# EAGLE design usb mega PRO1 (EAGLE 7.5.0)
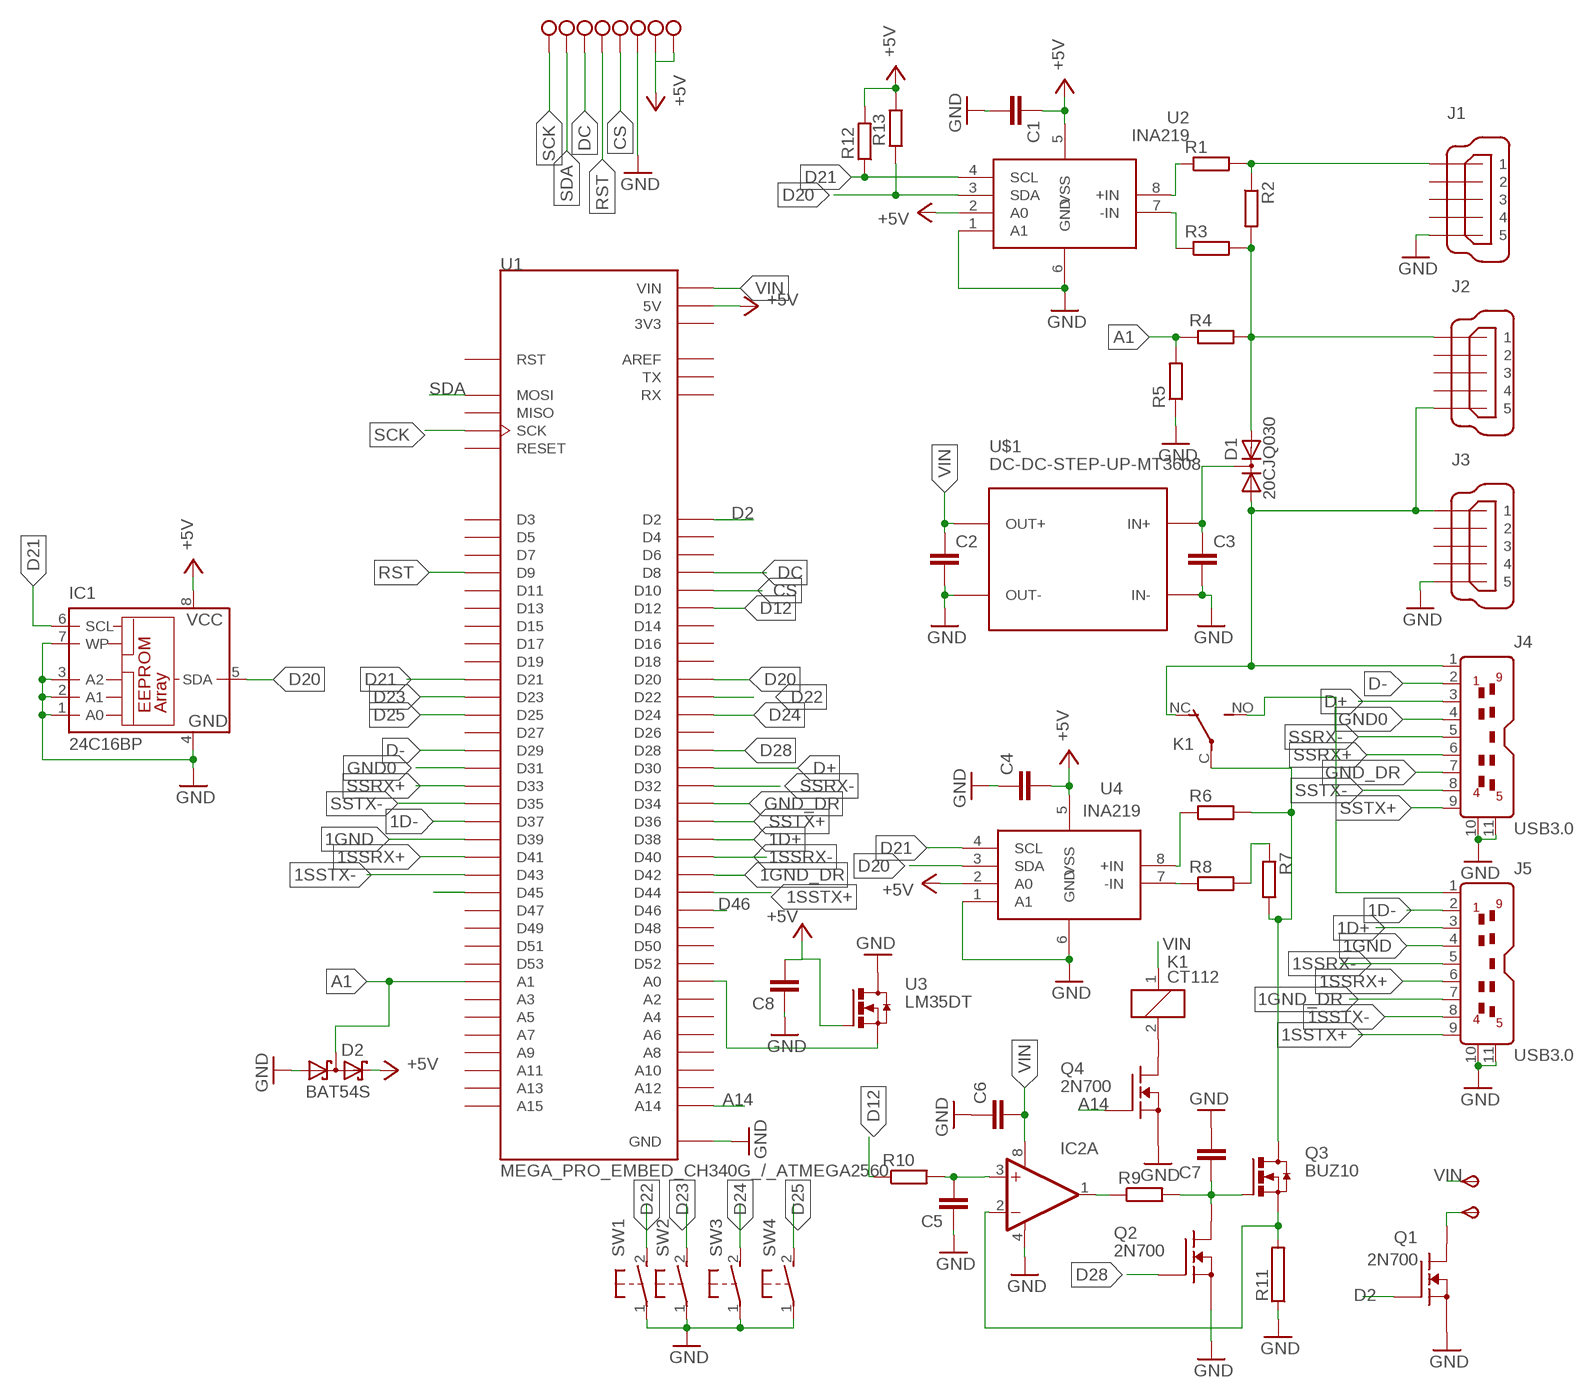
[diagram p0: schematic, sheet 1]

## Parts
C1  C-EUC0805  [C0805]
C2  C-EUC1206  [C1206]
C3  C-EUC1206  [C1206]
C4  C-EUC0805  [C0805]
C5  C-EUC0805  [C0805]
C6  C-EUC0805  [C0805]
C7  C-EUC0805  [C0805]
C8  C-EUC1206  [C1206]
D1  20CJQ030  [SOT223]
D2  BAT54S  [SOT23]
IC1  24C16BP  [DIL8]
IC2  OPA2658U  [SO08]
J1  MINI-USB_SHIELD5P2-32005-601  [32005-601]
J2  MINI-USB_SHIELD5P2-32005-601  [32005-601]
J3  MINI-USB_SHIELD5P2-32005-601  [32005-601]
J4  USB3.0  [USB3.0]
J5  USB3.0  [USB3.0]
K1  CT112  [CT-SLIM]
Q1  2N700  BSS138  [SOT23]
Q2  2N700  BSS138  [SOT23]
Q3  BUZ10  [TO220MIRROR]
Q4  2N700  BSS138  [SOT23]
R1  R-EU_R0805  [R0805]
R2  R-EU_R2010  [R2010]
R3  R-EU_R0805  [R0805]
R4  R-EU_R0805  [R0805]
R5  R-EU_R0805  [R0805]
R6  R-EU_R0805  [R0805]
R7  R-EU_R2010  [R2010]
R8  R-EU_R0805  [R0805]
R9  R-EU_R0805  [R0805]
R10  R-EU_R0805  [R0805]
R11  RAC01  [AC01]
R12  R-EU_R0805  [R0805]
R13  R-EU_R0805  [R0805]
SCK  TP2P2-38-17  [P2-38-17]
SCK1  TP2P2-38-17  [P2-38-17]
SCK2  TP2P2-38-17  [P2-38-17]
SCK3  TP2P2-38-17  [P2-38-17]
SW1  31-XX  [B3F-31XX]
SW2  31-XX  [B3F-31XX]
SW3  31-XX  [B3F-31XX]
SW4  31-XX  [B3F-31XX]
TP1  TPSPAD1-13  [P1-13]
TP2  TPSPAD1-13  [P1-13]
U1  MEGA_PRO_EMBED_CH340G_/_ATMEGA2560  [MODULE_MEGA_PRO_EMBED_CH340G_/_ATMEGA2560]
U2  INA219  [SO08]
U3  LM35DT  BUZ10  [TO220MIRROR]
U4  INA219  [SO08]
U$1  DC-DC-STEP-UP-MT3608  [DC-DC-STEP-UP-MT3608]

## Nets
1D+: J5.3 U1.D38
1D-: J5.2 U1.D37
1GND: J5.4 U1.D39
1GND_DR: J5.7 U1.D42
1SSRX+: J5.6 U1.D41
1SSRX-: J5.5 U1.D40
1SSTX+: J5.9 U1.D44
1SSTX-: J5.8 U1.D43
+5V: C1.1 C4.2 C8.2 D2.2(C2) IC1.8(VCC) R12.2 R13.2 SCK3.TP-1 SCK3.TP-2 U1.5V_1(5V) U1.5V_2(5V) U1.5V_3(5V) U2.2(A0) U2.5(VSS) U3.G U4.2(A0) U4.5(VSS)
A1: D2.3(C1A2) R4.1 R5.2 U1.A1
A14: Q4.3(G) U1.A14
CS: SCK2.TP-1 U1.D10
D2: Q1.3(G) U1.D2
D12: R10.1 U1.D12
D20: IC1.5(SDA) R13.1 U1.D20 U2.3(SDA) U4.3(SDA)
D21: IC1.6(SCL) R12.1 U1.D21 U2.4(SCL) U4.4(SCL)
D22: SW1.2(S) U1.D22
D23: SW2.2(S) U1.D23
D24: SW3.2(S) U1.D24
D25: SW4.2(S) U1.D25
D28: Q2.3(G) U1.D28
D45: U1.D45
D46: U1.D46
D+: J4.3 U1.D30
D-: J4.2 U1.D29
DC: SCK1.TP-1 U1.D8
GND: C1.2 C2.2 C3.2 C4.1 C5.1 C6.1 C7.2 C8.1 D2.1(A1) IC1.1(A0) IC1.2(A1) IC1.3(A2) IC1.4(GND) IC1.7(WP) IC2.4(A:V-) J1.5 J3.5 J4.10 J4.11 J5.10 J5.11 Q1.1(S) Q2.1(S) Q4.1(S) R5.1 R11.1 SCK2.TP-2 SW1.1(P) SW2.1(P) SW3.1(P) SW4.1(P) U1.GND_1(GND) U1.GND_2(GND) U1.GND_3(GND) U2.1(A1) U2.6(GND) U3.D U4.1(A1) U4.6(GND) U$1.IN- U$1.OUT-
GND0: J4.4 U1.D31
GND_DR: J4.7 U1.D34
N$1: R1.1 U2.8(+IN)
N$2: R3.1 U2.7(-IN)
N$3: J1.1 R1.2 R2.1
N$4: D1.3(A2) J2.1 R2.2 R3.2 R4.2
N$5: D1.1(A1) J2.5 J3.1 J4.1 K1.NC(2:O)
N$6: C3.1 D1.2(C) U$1.IN+
N$7: IC2.2(A:-IN) Q3.S R11.2
N$8: R6.1 U4.8(+IN)
N$9: R8.1 U4.7(-IN)
N$10: C5.2 IC2.3(A:+IN) R10.2
N$11: K1.C(2:P) Q3.D R6.2 R7.2
N$12: IC2.1(A:OUT) R9.1
N$13: C7.1 Q2.2(D) Q3.G R9.2
N$14: Q1.2(D) TP1.TP(PP)
N$15: R7.1 R8.2
N$16: K1.2 Q4.2(D)
N$17: U1.A0 U3.S
N$18: J5.1 K1.NO(2:S)
RST: SCK1.TP-2 U1.D9
SCK: SCK.TP-1 U1.SCK
SDA: SCK.TP-2 U1.MOSI
SSRX+: J4.6 U1.D33
SSRX-: J4.5 U1.D32
SSTX+: J4.9 U1.D36
SSTX-: J4.8 U1.D35
VIN: C2.1 C6.2 IC2.8(A:V+) K1.1 TP2.TP(PP) U1.VIN_1(VIN) U1.VIN_2(VIN) U$1.OUT+
Unconnected: IC2.5(B:+IN) IC2.6(B:-IN) IC2.7(B:OUT) J1.2 J1.3 J1.4 J1.M1(S1) J1.M2(S2) J2.2 J2.3 J2.4 J2.M1(S1) J2.M2(S2) J3.2 J3.3 J3.4 J3.M1(S1) J3.M2(S2) U1.A2 U1.A3 U1.A4 U1.A5 U1.A6 U1.A7 U1.A8 U1.A9 U1.A10 U1.A11 U1.A12 U1.A13 U1.A15 U1.AREF U1.D3 U1.D4 U1.D5 U1.D6 U1.D7 U1.D11 U1.D13 U1.D14 U1.D15 U1.D16 U1.D17 U1.D18 U1.D19 U1.D26 U1.D27 U1.D47 U1.D48 U1.D49 U1.D50 U1.D51 U1.D52 U1.D53 U1.MISO U1.RESET U1.RST U1.RX U1.TX

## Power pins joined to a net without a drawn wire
3V3: U1.3V3_1(3V3) U1.3V3_2(3V3)

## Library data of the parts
C1-C8 = rcl:C-EU: CAPACITOR, European symbol
D1 = diode:20CJQ030
D2 = diode:BAT54S: Schottky Diodes Pin connection corrected 2011-05-04 Source: Fairchild .. BAT54.pdf
IC1 = microchip:24*: Serial EEPROM I2C; MPN: AT24C16B-PU; OC_FARNELL: 1362650; OC_NEWARK: 50M3323
IC2 = burr-brown:OPA2658: Dual Wideband, Low Power, Current Feedback Operational Amplifier; OC_FARNELL: unknown; OC_NEWARK: unknown
J1-J3 = con-cypressindustries:MINI-USB_SHIELD5P2-: MINI USB-B R/A DIP 5pol. Source: www.cypressindustries.com; OC_FARNELL: unknown; OC_NEWARK: unknown
J4 J5 = con-cypressindustries:USB3.0
K1 = relay:CT112: ULTRA SMALL AUTOMOTIVE RELAY NAiS Slim 1c type en_ds_61205_0000.pdf; OC_FARNELL: unknown; OC_NEWARK: unknown
Q1 Q2 Q4 = transistor-fet:BSS138
Q3 U3 = transistor-power:BUZ10: BUZ10 MIRROR
R1-R10 R12 R13 = rcl:R-EU_: RESISTOR, European symbol
R11 = resistor-power:R: Power Resitor; OC_FARNELL: unknown; OC_NEWARK: unknown
SCK SCK1-SCK3 = testpad:TP2: Test pad
SW1-SW4 = switch-omron:31-XX: OMRON SWITCH; MPN: B3F-3100; OC_FARNELL: 959704; OC_NEWARK: 36M3582
TP1 TP2 = testpad:TPS: TEST PIN
U1 = MEGA_PRO_EMBED_CH340G___ATMEGA2560:MEGA_PRO_EMBED_CH340G_/_ATMEGA2560: Mega 2560 PRO (Embed) CH340G/ATmega2560-16AU Check availability; AVAILABILITY: Not in stock; MF: Robotdyn; MP: Mega Pro Embed CH340G / ATmega2560; PACKAGE: None; PRICE: None
U2 U4 = burr-brown:INA219: Bidirectional Current/Power Monitor With I2C Interface
U$1 = diy-modules:DC-DC-STEP-UP-MT3608: DC/DC Step-Up Regulator based on MT3608 chip MT3608 datasheet available here: https://www.olimex.com/Products/Breadboarding/BB-PWR-3608/resources/MT3608.pdf Click here to find device on ebay.com

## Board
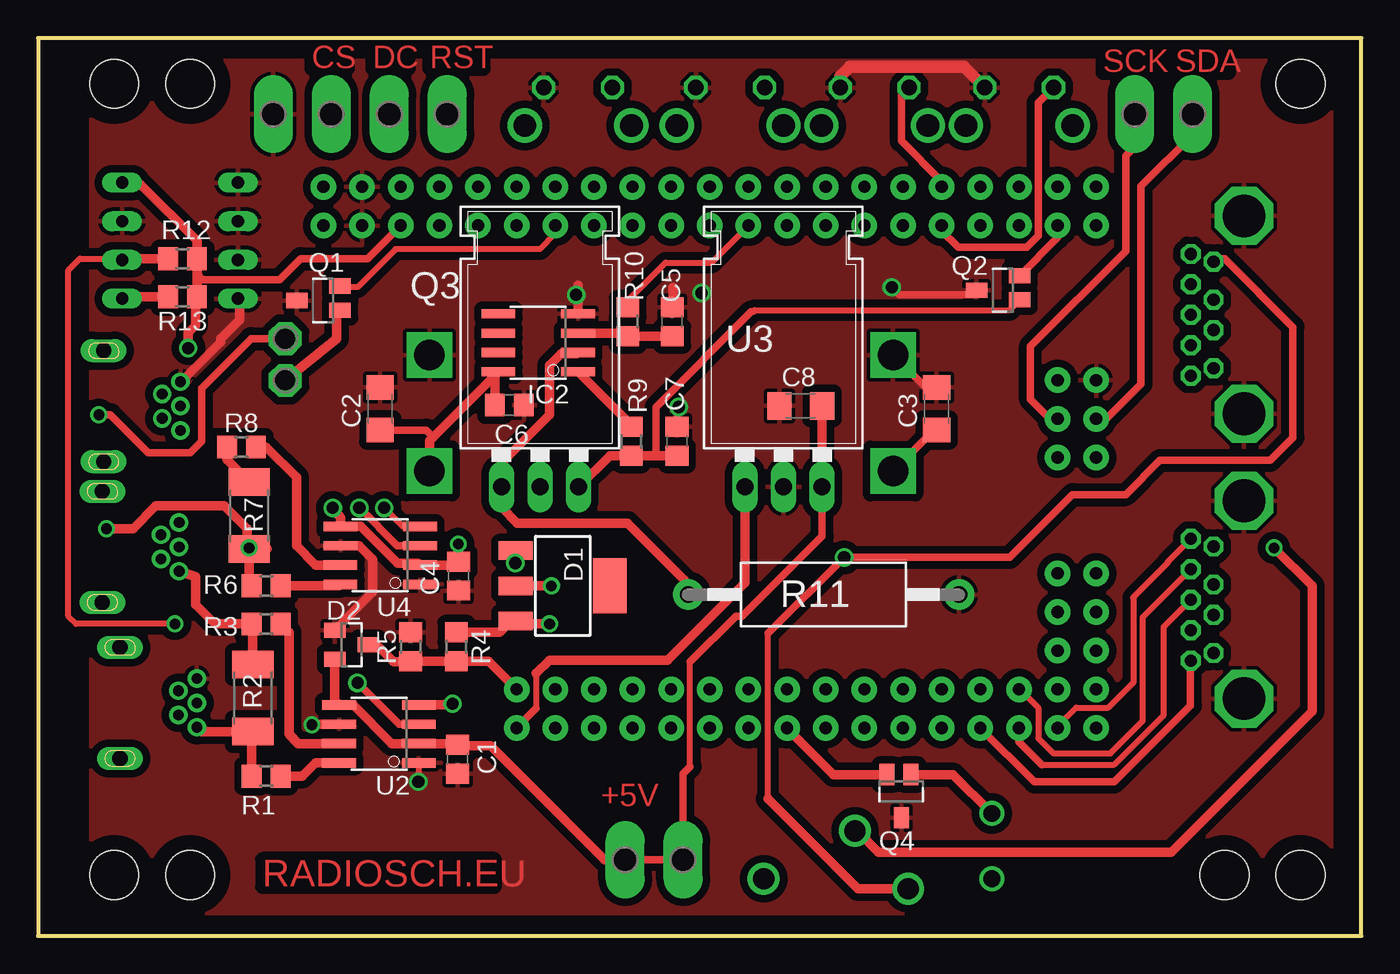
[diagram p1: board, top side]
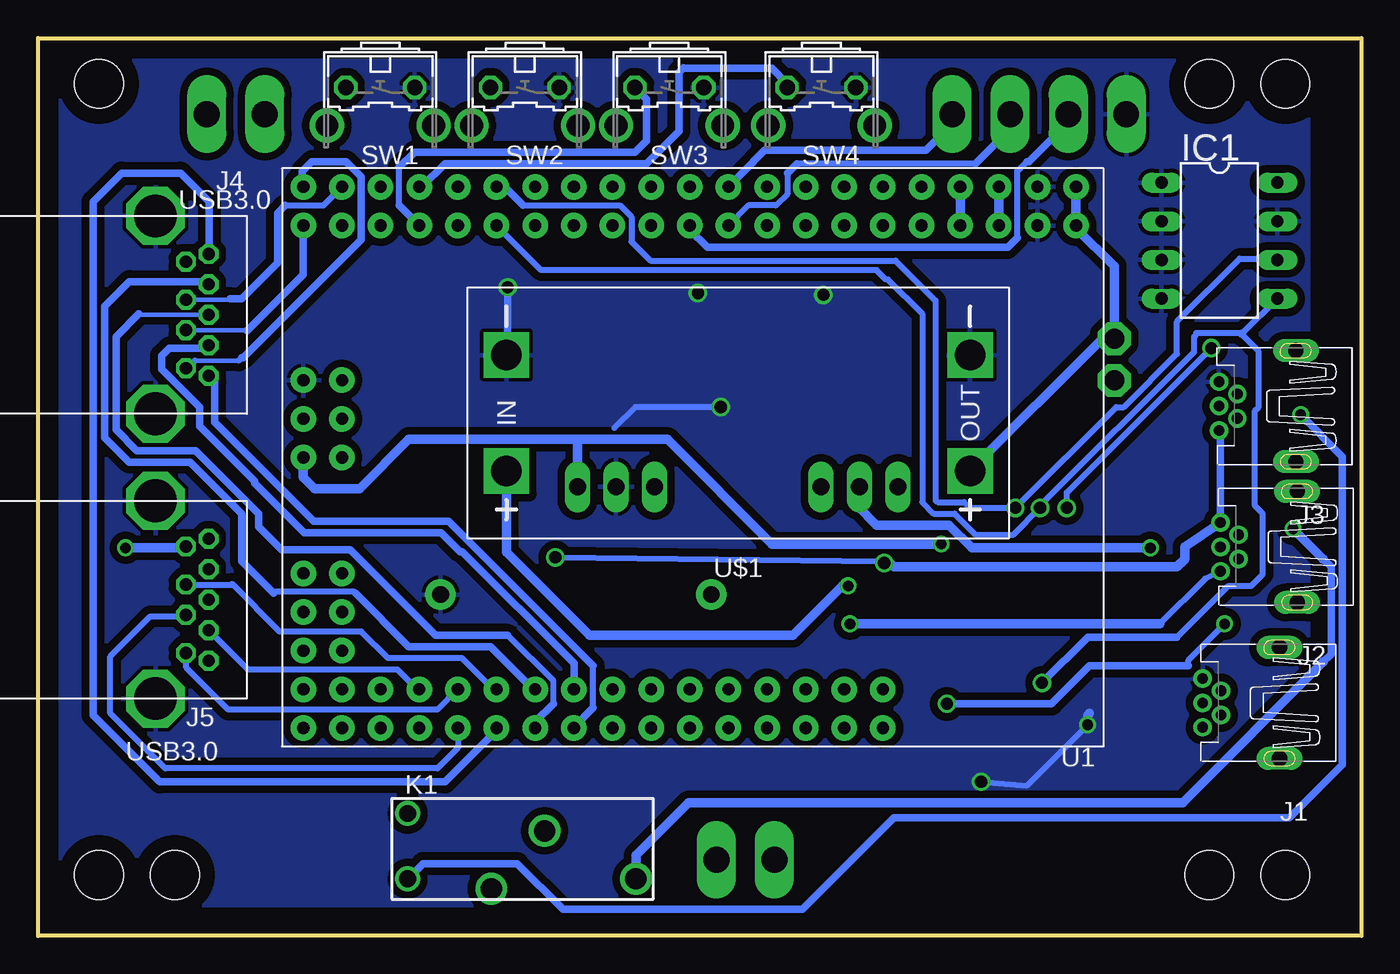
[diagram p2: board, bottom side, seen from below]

Size 87 x 59 mm. Coordinates in mm from the lower left corner, seen from the top.
Outline: 0,0 87,0 87,59 0,59 0,0
Copper layers (1*16): Top 0.035mm / dielectric 1.5mm / Bottom 0.035mm
Design rules "default *": minimum track width 10mil, minimum drill 24mil, track to track 6mil, track to pad 6mil, pad to pad 6mil, via to via 8mil, smd to smd 8mil, copper to edge 40mil, drill to drill 8mil, minimum pad ring 10mil, minimum via ring 8mil, stop-mask expansion 4mil, vias tented up to drill 0mil, thermal gap 10mil
Holes 3.2 mm at 5,56 83,56 5,4 83,4 10,56 10,4 78,4

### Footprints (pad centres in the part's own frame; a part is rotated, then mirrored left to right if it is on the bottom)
C0805 = smd 1.3 x 1.5: 1 -0.95,0; 2 0.95,0
C1206 = smd 1.6 x 1.8: 1 -1.4,0; 2 1.4,0
SOT223 = smd 1.219 x 2.235: 1 -2.311,-3.099; 2 0,-3.099; 3 2.311,-3.099 | smd 3.6 x 2.2: 4 0,3.099
SOT23 = smd 1 x 1.4: 1 -0.95,-1.1; 2 0.95,-1.1; 3 0,1.1
DIL8 = drill 0.813 long: 1 -3.81,-3.81; 2 -1.27,-3.81; 3 1.27,-3.81; 4 3.81,-3.81; 5 3.81,3.81; 6 1.27,3.81; 7 -1.27,3.81; 8 -3.81,3.81
SO08 = smd 0.61 x 2.21: 1 -1.905,-2.616; 2 -0.635,-2.616; 3 0.635,-2.616; 4 1.905,-2.616; 5 1.905,2.616; 6 0.635,2.616; 7 -0.635,2.616; 8 -1.905,2.616
32005-601 = drill 0.7 pad 1.016: 1 2.825,1.6; 2 1.625,0.8; 3 2.825,0; 4 1.625,-0.8; 5 2.825,-1.6 | drill 1 pad 1.422 long: M1 -2.225,3.65; M2 -2.225,-3.65
USB3.0 = drill 0.8 octagon: 1 0,0; 2 2.5,0; 3 4.5,0; 4 7,0; 5 7.5,1.5; 6 5.5,1.5; 7 3.5,1.5; 8 1.5,1.5; 9 -0.5,1.5 | drill 2.8 octagon: 10 -3,-2; 11 10,-2
CT-SLIM = drill 1.1: 1 -7.45,0; 2 -7.45,4.3 | drill 1.4: C 7.55,0; NC -1.95,-0.65; NO 1.55,3.15
SOT23' = smd 1 x 1.4: 1 0,1.735; 2 -0.632,-1.1; 3 0.95,-1.1
TO220MIRROR = drill 1.118 long: D 0,0; G 2.54,0; S -2.54,0
R0805 = smd 1.3 x 1.5: 1 -0.95,0; 2 0.95,0
R2010 = smd 1.8 x 2.7: 1 -2.2,0; 2 2.2,0
AC01 = drill 1.1 pad 2: 1 -8.9,0; 2 8.9,0
P2-38-17 = drill 1.702 pad 2.121 long: TP-1 -1.905,0; TP-2 1.905,0
B3F-31XX = drill 1.016 octagon: 1 -2.261,-1.245; 2 2.261,-1.245 | drill 1.499 pad 2.159: 3 -3.505,1.245; 4 3.505,1.245
P1-13 = drill 1.321 pad 2.159 octagon: TP 0,0
MODULE_MEGA_PRO_EMBED_CH340G_/_ATMEGA2560 = drill 0.8 pad 1.676: 3V3_1 -17.58,-17.78; 3V3_2 -17.58,-15.24; 5V_1 -20.12,-17.78; 5V_2 -20.12,-15.24; 5V_3 25.6,0; A0 -12.5,17.78; A1 -12.5,15.24; A2 -9.96,17.78; A3 -9.96,15.24; A4 -7.42,17.78; A5 -7.42,15.24; A6 -4.88,17.78; A7 -4.88,15.24; A8 -2.34,17.78; A9 -2.34,15.24; A10 0.2,17.78; A11 0.2,15.24; A12 2.74,17.78; A13 2.74,15.24; A14 5.28,17.78; A15 5.28,15.24; AREF -15.04,-15.24; D2 -9.96,-15.24; D3 -9.96,-17.78; D4 -7.42,-15.24; D5 -7.42,-17.78; D6 -4.88,-15.24; D7 -4.88,-17.78; D8 -2.34,-15.24; D9 -2.34,-17.78; D10 0.2,-15.24; D11 0.2,-17.78; D12 2.74,-15.24; D13 2.74,-17.78; D14 5.28,-15.24; D15 5.28,-17.78; D16 7.82,-15.24; D17 7.82,-17.78; D18 10.36,-15.24; D19 10.36,-17.78; D20 12.9,-15.24; D21 12.9,-17.78; D22 15.44,-15.24; D23 15.44,-17.78; D24 17.98,-15.24; D25 17.98,-17.78; D26 20.52,-15.24; D27 20.52,-17.78; D28 23.06,-15.24; D29 23.06,-17.78; D30 25.6,-15.24; D31 25.6,-17.78; D32 7.82,17.78; D33 7.82,15.24; D34 10.36,17.78; D35 10.36,15.24; D36 12.9,17.78; D37 12.9,15.24; D38 15.44,17.78; D39 15.44,15.24; D40 17.98,17.78; D41 17.98,15.24; D42 20.52,17.78; D43 20.52,15.24; D44 23.06,17.78; D45 23.06,15.24; D46 25.6,17.78; D47 25.6,15.24; D48 25.6,12.7; D49 23.06,12.7; D50 25.6,10.16; D51 23.06,10.16; D52 25.6,7.62; D53 23.06,7.62; GND_1 -22.66,-17.78; GND_2 -22.66,-15.24; GND_3 25.6,-5.08; MISO 23.06,0; MOSI 25.6,-2.54; RESET 23.06,-5.08; RST -15.04,-17.78; RX -12.5,-15.24; SCK 23.06,-2.54; TX -12.5,-17.78; VIN_1 -25.2,-17.78; VIN_2 -25.2,-15.24
DC-DC-STEP-UP-MT3608 = drill 2 pad 2.8 square: IN+ 15.24,3.81; IN- 15.24,-3.81; OUT+ -15.24,3.81; OUT- -15.24,-3.81

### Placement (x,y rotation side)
C1  27.59,11.61 270 top
C2  22.49,34.64 90 top
C3  59.07,34.64 90 top
C4  27.65,23.64 90 top
C5  41.69,40.36 270 top
C6  30.98,34.88 180 top
C7  42,32.5 90 top
C8  50.14,34.83 0 top
D1  34.5,23 270 top
D2  20.61,19.13 270 top
IC1  9.34,45.69 270 bottom
IC2  32.88,38.97 90 top
J1  7.61,15.31 180 bottom
J2  6.45,25.56 180 bottom
J3  6.54,34.81 180 bottom
J4  77.28,44.31 270 bottom
J5  77.28,25.59 270 bottom
K1  55.25,3.75 0 bottom
Q1  2N700  [SOT23']  18.75,41.75 90 top
Q2  2N700  [SOT23']  63.43,42.43 90 top
Q3  33,29.5 0 top
Q4  2N700  [SOT23']  56.75,9.5 180 top
R1  15,10.5 180 top
R2  14.12,15.62 90 top
R3  15,20.5 180 top
R4  27.5,19 90 top
R5  24.5,19 270 top
R6  15,23 180 top
R7  13.88,27.62 270 top
R8  13.38,32.12 180 top
R9  39,32.5 270 top
R10  38.77,40.36 270 top
R11  51.64,22.43 180 top
R12  9.5,44.5 0 top
R13  9.5,42 0 top
SCK  74,54 0 top
SCK1  25,54 0 top
SCK2  17.38,54 180 top
SCK3  40.5,5 0 top
SW1  64.5,54.5 180 bottom
SW2  55,54.5 180 bottom
SW3  45.5,54.5 180 bottom
SW4  35.5,54.5 180 bottom
TP1  16.25,36.5 0 top
TP2  16.25,39.25 0 top
U1  43.96,31.44 180 bottom
U2  22.41,13.27 90 top
U3  49,29.5 0 top
U4  22.5,25 90 top
U$1  40.97,34.36 180 bottom

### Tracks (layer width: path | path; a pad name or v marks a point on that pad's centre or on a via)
1D+
  Bottom 0.406: U1.D38 59.4,12.35 60.75,11 78.62,11 82.25,14.62 82.25,18.38 79.62,21 77.37,21 J5.3
1D-
  Bottom 0.406: U1.D37 57.08,16.2 59.12,18.25 64,18.25 65.75,20 71.12,20 74.25,23.12 74.28,23.09 J5.2
1GND
  Bottom 0.406: U1.D39 59.42,16.2 60.75,14.88 74.5,14.88 77.25,17.62 77.25,18.56 J5.4
1GND_DR
  Top 0.406: J5.7 74,20.31 74,14.5 70.75,11.25 66,11.25
  Top 0.5: U1.D42 64.48,12.77 66,11.25
1SSRX+
  Bottom 0.406: U1.D41 62.08,16.2 63.38,17.5 73.19,17.5 J5.6
1SSRX-
  Top 0.5: U1.D40 61.97,13.66 65.5,10.12 70.75,10.12 75.75,15.12 75.75,18.06 J5.5
1SSTX+
  Top 0.406: U1.D44 67.02,13.77 68.25,15 70.38,15 72,16.62 72,22.25 74.25,24.5 74.25,24.56 J5.9
1SSTX-
  Top 0.406: U1.D43 64.55,16.2 65.75,15 65.75,13 66.75,12 70.5,12 72.62,14.12 72.62,20.93 J5.8
3V3
  Bottom 0.61: U1.3V3_2 U1.3V3_1
+5V  (via drill 0.7, 0.8)
  Top 0.406: 42.88,11.12 42.88,18 | 10.45,42.67 R13.2
  Top 0.5: SCK3.TP-2 42.41,10.65 | 42.41,10.65 42.88,11.12 | 42.88,18 45.88,21 46.29,21 51.54,26.25 U3.G | SCK3.TP-2 SCK3.TP-1 | R13.2 10.75,42 | U1.5V_2 21.66,44.5 17.25,44.5 15.88,43.12 10.82,43.12 10.45,43.5 | SCK3.TP-2 42.41,10.65
  Top 0.61: SCK3.TP-1 37.25,5 29.75,12.5 27.65,12.5 C1.1 27.52,12.63 U2.2 25.02,12.62 23.25,12.62 20.7,15.18 U2.5 19.51,15.46 D2.2 | v27.62,25.75 27.65,25.73 C4.2 27.43,24.36 U4.2 24.98,24.5 23.62,24.5 21.22,26.91 U4.5 19.88,27.49 v19.38,28.12 | C8.2 U3.G | R13.2 10.38,41.92 10.38,40.12 9.88,39.62 v9.88,38.62 | 10.45,42.67 10.45,43.5 R12.2 10.45,45.67 6.75,49.38 5.65,49.38 IC1.8
  Bottom 0.406: v19.38,28.12 19.38,29.12 v9.88,38.62
  Bottom 0.61: U1.5V_3 69.56,30.12 68.81,29.38 65.88,29.38 62.62,32.62 51.54,32.62 | v27.62,25.75 38.75,25.75 45.62,32.62 51.54,32.62 | 51.54,32.62 U3.G | U1.5V_2 U1.5V_1
A1
  Top 0.61: D2.3 22.25,19.13 23.38,18 24.45,18 R5.2 R4.1 29.61,18.05 U1.A1
A14
  Top 0.61: Q4.3 52.3,10.6 U1.A14
CS
  Bottom 0.406: 22.62,45.88 22.62,50.25 22,50.88
  Bottom 0.5: U1.D10 44.16,46.41 43,45.25 23.25,45.25 22.62,45.88 | 22,50.88 21.88,50.88 19.25,53.5 19.25,53.97 SCK2.TP-1
D2
  Top 0.406: U1.D2 34,46.12 33,45.12 23.5,45.12 21,42.62 19.93,42.62 Q1.3
D12
  Top 0.406: R10.1 38.77,41.77 41.25,44.25 44.27,44.25 U1.D12
D20  (via drill 0.8)
  Top 0.406: U4.3 23.99,25.64
  Top 0.5: U4.3 23.61,25.64 v21.12,28.12 | U2.3 23.72,13.9 v21,16.62
  Top 0.61: R13.1 5.65,42 IC1.5
  Bottom 0.406: 10.88,39.62 10.75,39.62 | 10.75,39.62 7.79,39.62 IC1.5 | 10.75,39.62 11,39.38 11,38.38 21.12,28.25 v21.12,28.12 22.88,26.38 25.38,26.38 26.75,27.75 28.12,27.75 28.88,28.5 28.88,40.88 31.12,43.12 31.25,43.12 31.88,43.75 53.93,43.75 U1.D20 | 12.12,19.62 8.75,23 7.25,23 6.5,23.75 6.5,27.75 7,28.25 7,34.5 6.75,34.75 6.75,38.41 7.88,39.53
  Bottom 0.5: v21,16.62 18,19.62 12.12,19.62 | 7.88,39.53 7.79,39.62
D21  (via drill 0.7, 0.8)
  Top 0.406: U4.4 23.97,26.91 v22.75,28.12 | v9,20.5 2.5,20.5 2,21 2,43.75 2.75,44.5 5.45,44.5 IC1.6
  Top 0.61: R12.1 5.61,44.5 IC1.6 | U2.4 27.18,15.18 v27.25,15.25
  Bottom 0.406: IC1.6 5.61,44.5 8,44.5 12.12,40.38 12.12,38.25 15.62,34.75 16.12,34.75 v22.75,28.12 25.75,28.12 26.12,28.5 27.88,28.5 28,28.62 28,41.75 30.62,44.38 46.75,44.38 48,45.62 48,47.25 48.75,48 55.12,48 | 11.38,17.75 11.38,18.12 v9,20.5
  Bottom 0.5: U1.D21 56.34,49.22 55.12,48 | v27.25,15.25 20.38,15.25 17.88,17.75 11.38,17.75
D22
  Top 0.5: U1.D22 59.4,46.35 60.5,45.25 65,45.25 65.75,46 65.75,54.73 SW1.2
D23
  Top 0.5: U1.D23 59.4,49.6 56.75,52.25 56.75,55.23 SW2.2
D24
  Bottom 0.406: 63.25,48 63.25,50.5
  Bottom 0.5: U1.D24 63.25,48 | 63.25,50.5 62.25,51.5 47.75,51.5 47,52.25 47,54.98 SW3.2
D25
  Bottom 0.5: U1.D25 61.78,49.22 60.25,50.75 47,50.75 44.88,52.88 44.88,56.75 44.56,57.06 44.5,57 38.75,57 37.76,56.01 SW4.2
D28
  Top 0.5: U1.D28 67.02,45.87 Q2.3
D+
  Bottom 0.305: J4.3 73.31,39.81
  Bottom 0.406: 73.31,39.81 73.25,39.75
  Bottom 0.5: U1.D30 69.56,43.44 73.25,39.75
D-
  Bottom 0.305: J4.2 74.44,41.81 74.38,41.88
  Bottom 0.406: 70.75,48 68.24,48 U1.D29
  Bottom 0.5: 74.38,41.88 73.62,41.88 71.25,44.25 71.25,47.5 70.75,48
DC
  Bottom 0.406: 25.38,50.75 37.12,50.75 | 37.75,50.12 37.75,48.75 38.5,48 40.3,48 U1.D8
  Bottom 0.5: SCK1.TP-1 23.09,53.03 25.38,50.75 | 37.12,50.75 37.75,50.12
GND  (via drill 0.7, 0.8)
  Top 0.406: C7.2 42,34.62 v42.12,34.75 | U2.1 25.03,9.9 v25,10.12
  Top 0.5: C3.2 58.34,36.04 U$1.IN- | Q2.1 61.7,42.2 61.62,42.12 56.62,42.12 v56.12,42.62
  Top 0.61: U2.6 18.03,13.9 v18,13.88 | IC2.4 35.5,42.75 v35.38,42.12 | 41.75,42.62 41.75,41.37 C5.1 | U4.6 21.11,25.64 22,24.75 22,22.57 D2.1 | J3.5 9.41,36.41 12,39 12,39.25 13.25,40.5 13.25,41.78 IC1.4
  Top 0.813: SW2.1 52.74,56.49 53.38,57.12 60.86,57.12 SW1.1
  Bottom 0.406: v42.12,34.75 47.75,34.75 49.12,33.38 | v25,10.12 22,9.88 v18,13.88
  Bottom 0.5: v56.12,42.62 56.12,38.26 U$1.IN-
  Bottom 0.61: v18,13.88 18,14.5 17.88,14.62
  other vias: 43.62,42.25
  pour Top (isolate 0.5): 3.5,57.5 85,57.5 85,1.5 3.5,1.5
  pour Bottom (isolate 0.5): 3.5,57.5 85.5,57.5 85.5,2 3.5,2
GND0
  Bottom 0.305: 76.67,37.8 73.83,37.8
  Bottom 0.406: J4.4 77.17,37.31 76.67,37.8 | 73.83,37.8 73.62,38
  Bottom 0.5: 73.62,38 73.5,38 65.75,45.75 65.75,49.88 66.75,50.88 69,50.88 69.62,50.25 69.62,49.28 U1.D31
GND_DR
  Bottom 0.305: J4.7 80.31,40.81 80.38,40.88
  Bottom 0.406: 53.12,15.25 53.12,16.75 56.12,19.75
  Bottom 0.5: U1.D34 54.32,14.05 53.12,15.25 | 56.12,19.75 60.88,19.75 66.5,25.38 71,25.38 72.5,26.88 72.5,27.75 76.62,31.88 80.5,31.88 81.88,33.25 81.88,39.38 80.38,40.88
N$1
  Top 0.61: R1.1 17.38,10.5 18.25,11.38 U2.8
N$2
  Top 0.61: U2.7 17.12,12.63 16.5,13.25 16.5,19.95 R3.1
N$3
  Top 0.61: J1.1 10.72,13.43 R2.1 14.05,13.35 R1.2
N$4  (via drill 0.7)
  Top 0.61: R2.2 14.12,20.43 R3.2 11.62,20.5 10.38,21.75 10.38,23.61 J2.1 | v33.62,20.5 31.59,20.5 D1.3 31.21,20.5 30.88,20.5 30.32,19.95 R4.2
  Bottom 0.406: J2.1 10.28,23.48 13.25,20.5
  Bottom 0.61: 13.25,20.5 v33.62,20.5
N$5  (via drill 0.8)
  Top 0.406: 48,9 48,19.88
  Top 0.5: J4.1 77.47,44.5 78,44.5 82.5,40 82.5,32.75 81,31.25 73.75,31.25 71.5,29 68,29 63.88,24.88 v53,24.88 48,19.88
  Top 0.61: D1.1 31.4,24.53 v31.38,24.5 | K1.NC 53.9,3.1 48,9
  Bottom 0.406: v53,24.88 31.5,24.62 v31.38,24.5
  Bottom 0.5: J2.5 9.28,33.12 J3.1
  Bottom 0.61: v31.38,24.5 31,24.5 30.75,24.25 12.12,24.25 11.62,24.75 11.62,25.56 J2.5
N$6  (via drill 0.7)
  Top 0.5: C3.1 58.9,33.24 U$1.IN+
  Top 0.61: D1.2 v33.75,23
  Bottom 0.61: v33.75,23 34.12,23 37.38,19.75 50.75,19.75 56.21,25.21 U$1.IN+
N$7
  Top 0.61: R11.2 42.5,22.67 42.5,23.38 38.75,27.12 31.5,27.12 30.46,28.16 Q3.S 30.46,31.09 33.62,34.25 33.62,37.5 34.38,38.25 35.41,38.25 IC2.2
N$8
  Top 0.61: R6.1 19.79,23 U4.8
N$9
  Top 0.61: U4.7 18.26,24.36 17,25.62 17,30.12 15,32.12 R8.1
N$10
  Top 0.61: IC2.3 38.58,39.6 R10.2 C5.2
N$11  (via drill 0.7)
  Top 0.61: R6.2 13.88,23.18 R7.2 15.05,25.43 v13.88,25.5 13.75,25.62 13.75,26.75 12.25,28.25 7.75,28.25 6.25,26.75 v4.5,26.75
  Bottom 0.5: 2.5,18 2,18.5 2,24.25 2.5,24.75
  Bottom 0.61: Q3.D 33.12,29.38 33.12,28.25 31.88,27 27.12,27 25.62,25.5 v13.88,25.5 | 2.5,18 11.75,8.75 44.25,8.75 47.7,5.3 K1.C | 2.5,24.75 v4.5,26.75
N$12
  Top 0.61: R9.1 39,33.56 IC2.1
N$13
  Top 0.406: 46.88,41 47,41 47.12,41.12 63.86,41.12 Q2.2
  Top 0.5: 46.88,41 40.62,34.75 40.62,31.8 40.38,31.55
  Top 0.61: C7.1 40.38,31.55 R9.2 37.59,31.55 Q3.G
N$14
  Top 0.61: TP1.TP 19.62,39.25 19.62,40.89 Q1.2
N$15
  Top 0.61: R8.2 12.43,31.27 R7.1
N$16
  Top 0.61: Q4.2 60.15,10.6 K1.2
N$17
  Top 0.406: 32.75,17.25 32.75,14.95
  Top 0.5: 32.75,14.95 U1.A0
  Top 0.61: U3.S 46.46,23.21 41.38,18.12 33.62,18.12 32.75,17.25
N$18  (via drill 0.7)
  Top 0.61: K1.NO 53.85,6.9 55.25,5.5 74.5,5.5 83.75,14.75 83.75,23 v81.25,25.5
  Bottom 0.61: v81.25,25.5 77.37,25.5 J5.1
RST
  Bottom 0.5: SCK1.TP-2 26.91,53.34 28.62,51.62 39.25,51.62 39.97,50.91 39.97,50.88 U1.D9
SCK
  Top 0.5: U1.SCK 66.52,33.98 65.25,35.25 65.25,38.75 71.5,45 71.5,51.25 72,51.75 72,53.91 SCK.TP-1
SDA
  Top 0.5: U1.MOSI 70.23,33.98 72.5,36.25 72.5,49.25 76,52.75 76,54.16 SCK.TP-2
SSRX+
  Bottom 0.5: U1.D33 51.78,17.91 59.12,25.25 59.25,25.25 60.5,26.5 69.5,26.5 72.75,29.75 72.75,29.88 76.38,33.5 76.38,34.75 78.88,37.25 78.88,38.12 78.38,38.62 75.97,38.62 J4.6
SSRX-
  Bottom 0.406: 50.5,15 50.5,17.75
  Bottom 0.5: U1.D32 51.78,13.72 50.5,15 | 50.5,17.75 60,27.25 68.88,27.25 75.38,33.75 75.38,36.41 J4.5
SSTX+
  Bottom 0.5: U1.D36 56.86,13.52 60.25,10.12 79,10.12 83.38,14.5 83.38,48.25 81.5,50.12 77.62,50.12 75.75,48.25 75.75,44.84 J4.9
SSTX-
  Bottom 0.406: 66.12,22.5 66.25,22.62 71.38,22.62 71.5,22.5
  Bottom 0.5: U1.D35 54.45,16.2 57.25,19 62.62,19 66.12,22.5 | 71.5,22.5 73.62,24.62 73.62,27.75 77,31.12 81,31.12 82.62,32.75 82.62,41.38 81,43 75.97,43 J4.8
VIN  (via drill 0.7)
  Top 0.5: C2.1 25.51,33.24 25.97,32.78 | v4,34.25 4.75,34.25 7.25,31.75 10,31.75 10.75,32.5 10.75,36 14,39.25 TP2.TP
  Top 0.61: U$1.OUT+ 25.73,32.53 25.97,32.78 IC2.8 30.04,36.84 C6.2
  Bottom 0.5: 62.7,3.2 K1.1 61.7,4.75 55.5,4.75 52.5,1.75 36.75,1.75 30.75,7.75 4.75,7.75 1.25,11.25 1.25,31.5 v4,34.25
  Bottom 0.61: U$1.OUT+ 17.03,39.25 TP2.TP 16.25,44 18.76,46.51 U1.VIN_2 U1.VIN_1

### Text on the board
Top: CS | DC | RST | SCK | SDA | +5V | RADIOSCH.EU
